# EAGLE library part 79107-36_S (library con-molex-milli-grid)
RECEPTACAL
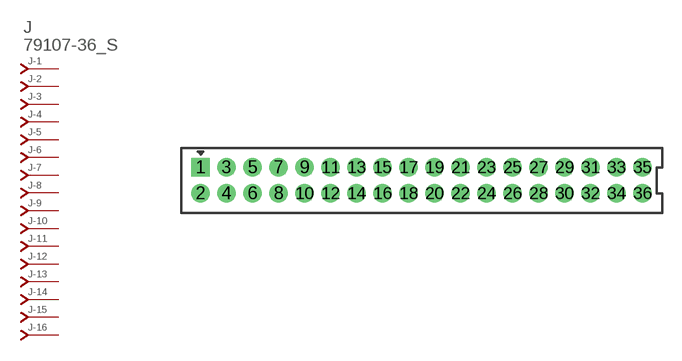
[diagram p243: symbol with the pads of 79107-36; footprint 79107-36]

Designator prefix J; gates -1=J-NV -2=J-N -3=J-N -4=J-N -5=J-N -6=J-N -7=J-N -8=J-N -9=J-N -10=J-N -11=J-N -12=J-N -13=J-N -14=J-N -15=J-N -16=J-N -17=J-N -18=J-N -19=J-N -20=J-N -21=J-N -22=J-N -23=J-N -24=J-N -25=J-N -26=J-N -27=J-N -28=J-N -29=J-N -30=J-N -31=J-N -32=J-N -33=J-N -34=J-N -35=J-N -36=J-N

## 79107-36_S  [79107-36]
1  -1:J  pas
2  -2:J  pas
3  -3:J  pas
4  -4:J  pas
5  -5:J  pas
6  -6:J  pas
7  -7:J  pas
8  -8:J  pas
9  -9:J  pas
10  -10:J  pas
11  -11:J  pas
12  -12:J  pas
13  -13:J  pas
14  -14:J  pas
15  -15:J  pas
16  -16:J  pas
17  -17:J  pas
18  -18:J  pas
19  -19:J  pas
20  -20:J  pas
21  -21:J  pas
22  -22:J  pas
23  -23:J  pas
24  -24:J  pas
25  -25:J  pas
26  -26:J  pas
27  -27:J  pas
28  -28:J  pas
29  -29:J  pas
30  -30:J  pas
31  -31:J  pas
32  -32:J  pas
33  -33:J  pas
34  -34:J  pas
35  -35:J  pas
36  -36:J  pas

## Footprint 79107-36 (pad centres in mm)
RECEPTACAL Dual Row, Vertical, Through-Hole
drill 0.914 square: 1 -17,1
drill 0.914: 2 -17,-1; 3 -15,1; 4 -15,-1; 5 -13,1; 6 -13,-1; 7 -11,1; 8 -11,-1; 9 -9,1; 10 -9,-1; 11 -7,1; 12 -7,-1; 13 -5,1; 14 -5,-1; 15 -3,1; 16 -3,-1; 17 -1,1; 18 -1,-1; 19 1,1; 20 1,-1; 21 3,1; 22 3,-1; 23 5,1; 24 5,-1; 25 7,1; 26 7,-1; 27 9,1; 28 9,-1; 29 11,1; 30 11,-1; 31 13,1; 32 13,-1; 33 15,1; 34 15,-1; 35 17,1; 36 17,-1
